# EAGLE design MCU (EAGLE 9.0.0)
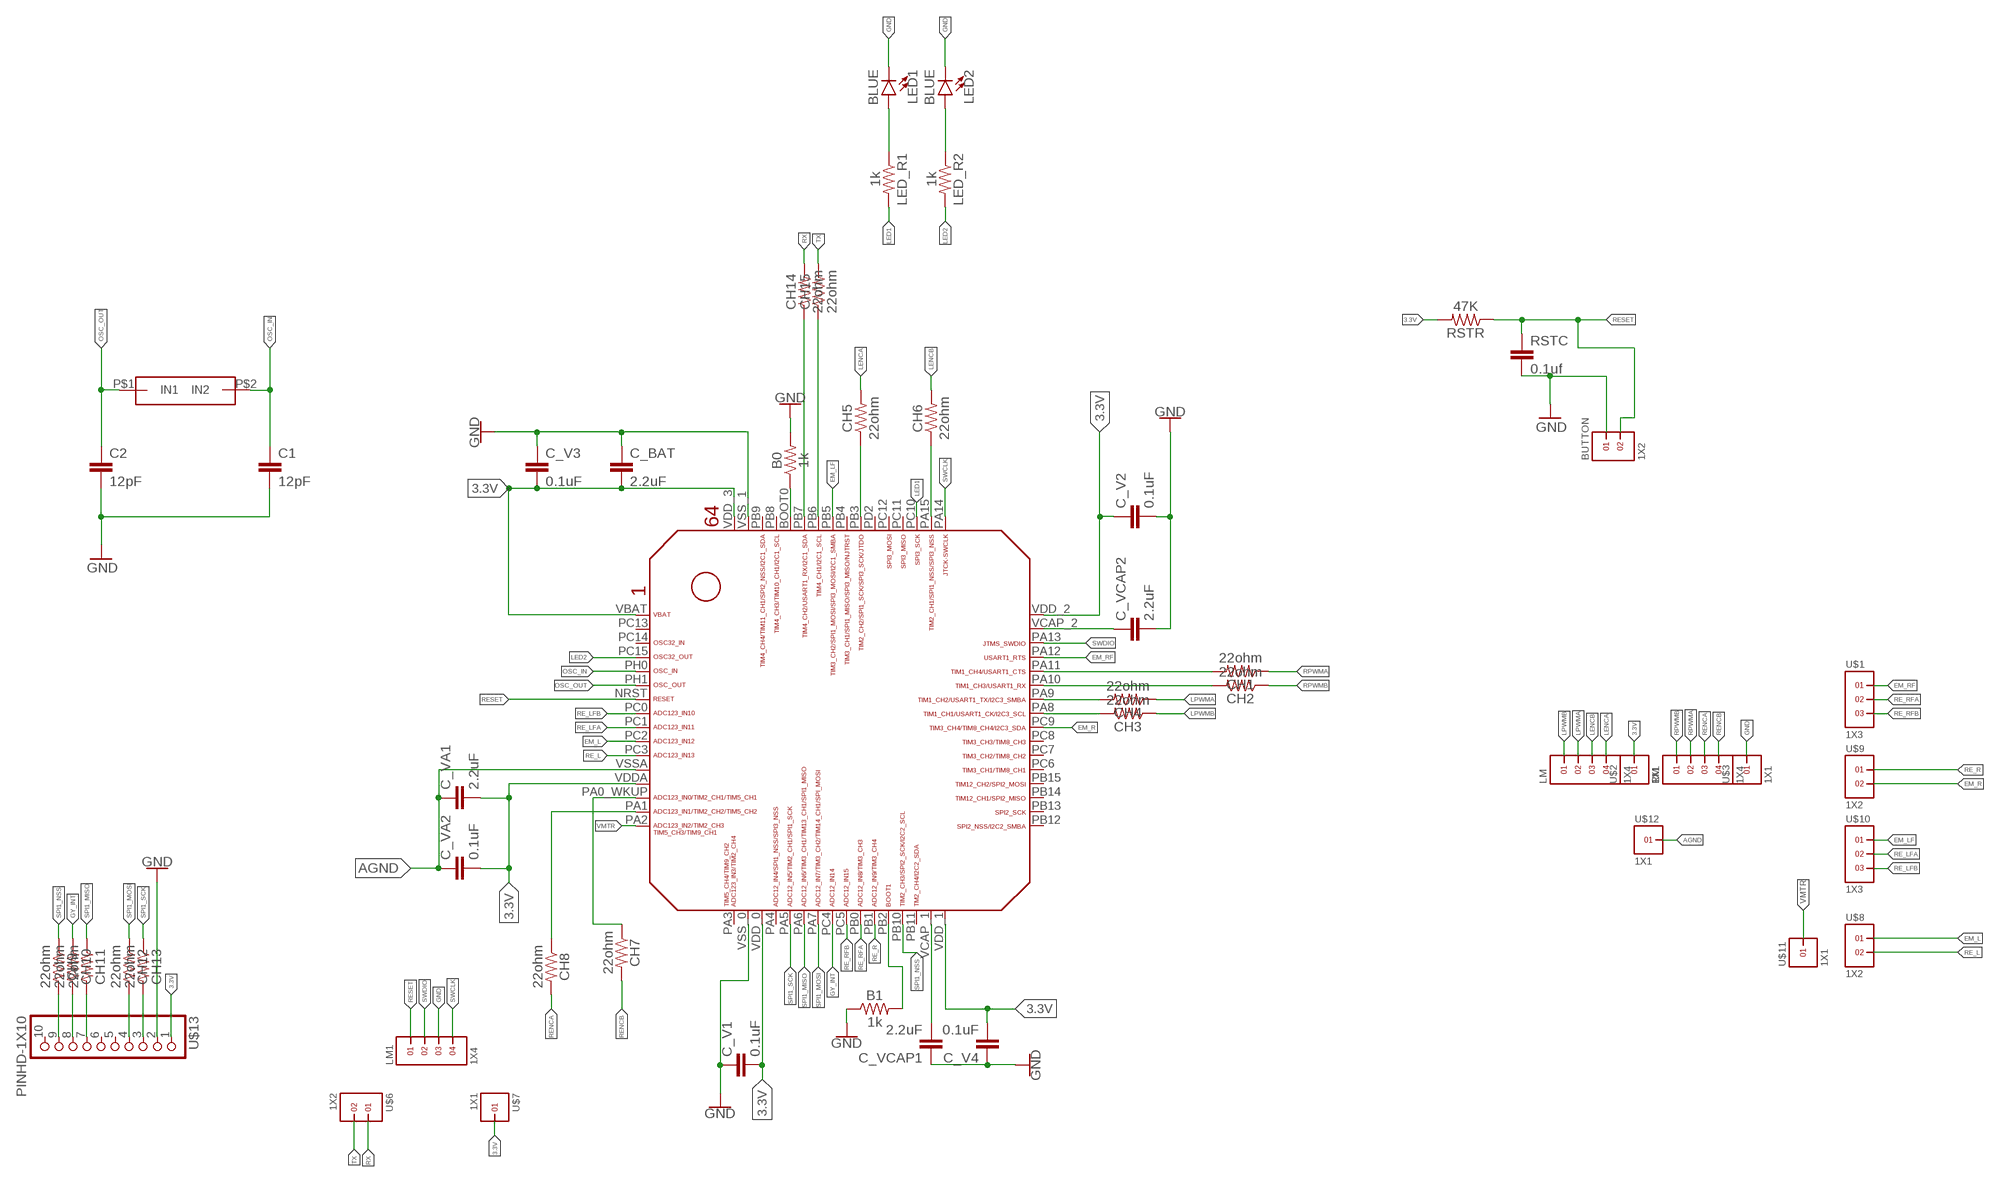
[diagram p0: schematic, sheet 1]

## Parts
B0  1k  0.75OHM-0805-1/4W-1%  [0805]
B1  1k  0.75OHM-0805-1/4W-1%  [0805]
BUTTON  1X2  [1X2]
C1  12pF  22PF-0603-50V-5%  [0603]
C2  12pF  22PF-0603-50V-5%  [0603]
C_BAT  2.2uF  22UF-0805-6.3V-20%  [0805]
C_V1  0.1uF  22UF-0805-6.3V-20%  [0805]
C_V2  0.1uF  22UF-0805-6.3V-20%  [0805]
C_V3  0.1uF  22UF-0805-6.3V-20%  [0805]
C_V4  0.1uF  22UF-0805-6.3V-20%  [0805]
C_VA1  2.2uF  22UF-0805-6.3V-20%  [0805]
C_VA2  0.1uF  22UF-0805-6.3V-20%  [0805]
C_VCAP1  2.2uF  22UF-0805-6.3V-20%  [0805]
C_VCAP2  2.2uF  22UF-0805-6.3V-20%  [0805]
CH1  22ohm  0.75OHM-0805-1/4W-1%  [0805]
CH2  22ohm  0.75OHM-0805-1/4W-1%  [0805]
CH3  22ohm  0.75OHM-0805-1/4W-1%  [0805]
CH4  22ohm  0.75OHM-0805-1/4W-1%  [0805]
CH5  22ohm  0.75OHM-0805-1/4W-1%  [0805]
CH6  22ohm  0.75OHM-0805-1/4W-1%  [0805]
CH7  22ohm  0.75OHM-0805-1/4W-1%  [0805]
CH8  22ohm  0.75OHM-0805-1/4W-1%  [0805]
CH9  22ohm  0.75OHM-0805-1/4W-1%  [0805]
CH10  22ohm  0.75OHM-0805-1/4W-1%  [0805]
CH11  22ohm  0.75OHM-0805-1/4W-1%  [0805]
CH12  22ohm  0.75OHM-0805-1/4W-1%  [0805]
CH13  22ohm  0.75OHM-0805-1/4W-1%  [0805]
CH14  22ohm  0.75OHM-0805-1/4W-1%  [0805]
CH15  22ohm  0.75OHM-0805-1/4W-1%  [0805]
LED1  BLUE  LED-BLUE1206  [LED-1206]
LED2  BLUE  LED-BLUE1206  [LED-1206]
LED_R1  1k  0.75OHM-0805-1/4W-1%  [0805]
LED_R2  1k  0.75OHM-0805-1/4W-1%  [0805]
LM  1X4  [1X4]
LM1  1X4  [1X4]
RM  1X4  [1X4]
RSTC  0.1uf  22UF-0805-6.3V-20%  [0805]
RSTR  47K  0.75OHM-0805-1/4W-1%  [0805]
U$1  1X3  [1X3]
U$2  1X1  [1X1]
U$3  1X1  [1X1]
U$4  STM32F405/415_LQFP64  [STM32F405/415_LQFP64]
U$5  OSC  [OSC]
U$6  1X2  [1X2]
U$7  1X1  [1X1]
U$8  1X2  [1X2]
U$9  1X2  [1X2]
U$10  1X3  [1X3]
U$11  1X1  [1X1]
U$12  1X1  [1X1]
U$13  PINHD-1X10  [1X10-BIG]

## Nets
3.3V: C_BAT.2 C_V1.2 C_V2.1 C_V3.2 C_V4.2 C_VA1.2 C_VA2.2 RSTR.2 U$2.1 U$4.VBAT U$4.VDD_0 U$4.VDD_1 U$4.VDD_2 U$4.VDD_3 U$4.VDDA U$7.1 U$13.1
AGND: C_VA1.1 C_VA2.1 U$4.VSSA U$12.1
EM_L: U$4.PC2 U$8.1
EM_LF: U$4.PB5 U$10.1
EM_R: U$4.PC9 U$9.2
EM_RF: U$1.1 U$4.PA12
GND: B0.2 B1.1 BUTTON.1 C1.2 C2.2 C_BAT.1 C_V1.1 C_V2.2 C_V3.1 C_V4.1 C_VCAP1.1 C_VCAP2.2 LED1.C LED2.C LM1.3 RSTC.2 U$3.1 U$4.VSS_0 U$4.VSS_1 U$13.2
GY_INT: CH10.1 U$4.PC4
INT: CH10.2 U$13.8
LED1: LED_R1.2 U$4.PC10
LED2: LED_R2.2 U$4.PC15
LENCA: CH5.2 LM.4
LENCB: CH6.2 LM.3
LPWMA: CH4.1 LM.2
LPWMB: CH3.1 LM.1
MISO: CH11.2 U$13.7
MOSI: CH12.2 U$13.4
N$1: CH3.2 U$4.PA8
N$2: CH4.2 U$4.PA9
N$3: CH1.2 U$4.PA11
N$4: CH2.2 U$4.PA10
N$5: CH6.1 U$4.PA15
N$6: CH5.1 U$4.PB3
N$7: CH7.1 U$4.PA0_WKUP(PA0_AKUP)
N$8: CH8.1 U$4.PA1
N$9: B1.2 U$4.PB2
N$10: B0.1 U$4.BOOT0
N$11: CH14.1 U$4.PB7
N$12: CH15.1 U$4.PB6
N$13: LED2.A LED_R2.1
N$14: LED1.A LED_R1.1
NSS: CH9.2 U$13.9
OSC_IN: C1.1 U$4.PH0 U$5.P$2(IN2)
OSC_OUT: C2.1 U$4.PH1 U$5.P$1(IN1)
RE_L: U$4.PC3 U$8.2
RE_LFA: U$4.PC1 U$10.2
RE_LFB: U$4.PC0 U$10.3
RE_R: U$4.PB1 U$9.1
RE_RFA: U$1.2 U$4.PB0
RE_RFB: U$1.3 U$4.PC5
RENCA: CH8.2 RM.3
RENCB: CH7.2 RM.4
RESET: BUTTON.2 LM1.1 RSTC.1 RSTR.1 U$4.NRST
RPWMA: CH1.1 RM.2
RPWMB: CH2.1 RM.1
RX: CH14.2 U$6.1
SCK: CH13.2 U$13.3
SPI1_MISO: CH11.1 U$4.PA6
SPI1_MOSI: CH12.1 U$4.PA7
SPI1_NSS: CH9.1 U$4.PB10
SPI1_SCK: CH13.1 U$4.PA5
SWCLK: LM1.4 U$4.PA14
SWDIO: LM1.2 U$4.PA13
TX: CH15.2 U$6.2
VCAP_1: C_VCAP1.2 U$4.VCAP_1
VCAP_2: C_VCAP2.1 U$4.VCAP_2
VMTR: U$4.PA2 U$11.1
Unconnected: U$4.PA3 U$4.PA4 U$4.PB4 U$4.PB8 U$4.PB9 U$4.PB11 U$4.PB12 U$4.PB13 U$4.PB14 U$4.PB15 U$4.PC6 U$4.PC7 U$4.PC8 U$4.PC11 U$4.PC12 U$4.PC13 U$4.PC14 U$4.PD2 U$13.5 U$13.6 U$13.10

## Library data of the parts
B0 B1 CH1-CH15 LED_R1 LED_R2 RSTR = SparkFun-Resistors:0.75OHM: 0.75Ω resistor; PROD_ID: RES-08474; VALUE: 0.75
BUTTON U$6 U$8 U$9 = headers(2mm):1X2
C1 C2 = SparkFun-Capacitors:22PF: 22pF ceramic capacitors; PROD_ID: CAP-07876; VALUE: 22pF
C_BAT C_V1-C_V4 C_VA1 C_VA2 C_VCAP1 C_VCAP2 RSTC = SparkFun-Capacitors:22UF: 22µF ceramic capacitors; PROD_ID: CAP-08402; VALUE: 22uF
LED1 LED2 = SparkFun-LED:LED-BLUE: Blue SMD LED; PROD_ID: DIO-09911
LM LM1 RM = headers(2mm):1X4
U$1 U$10 = headers(2mm):1X3
U$2 U$3 U$7 U$11 U$12 = headers(2mm):1X1
U$4 = STM32F405RG:STM32F405/415_LQFP64
U$5 = Cristal Oscillator:OSC
U$13 = adafruit:PINHD-1X10: Pin header 1x10 0.1" spacing With round pins

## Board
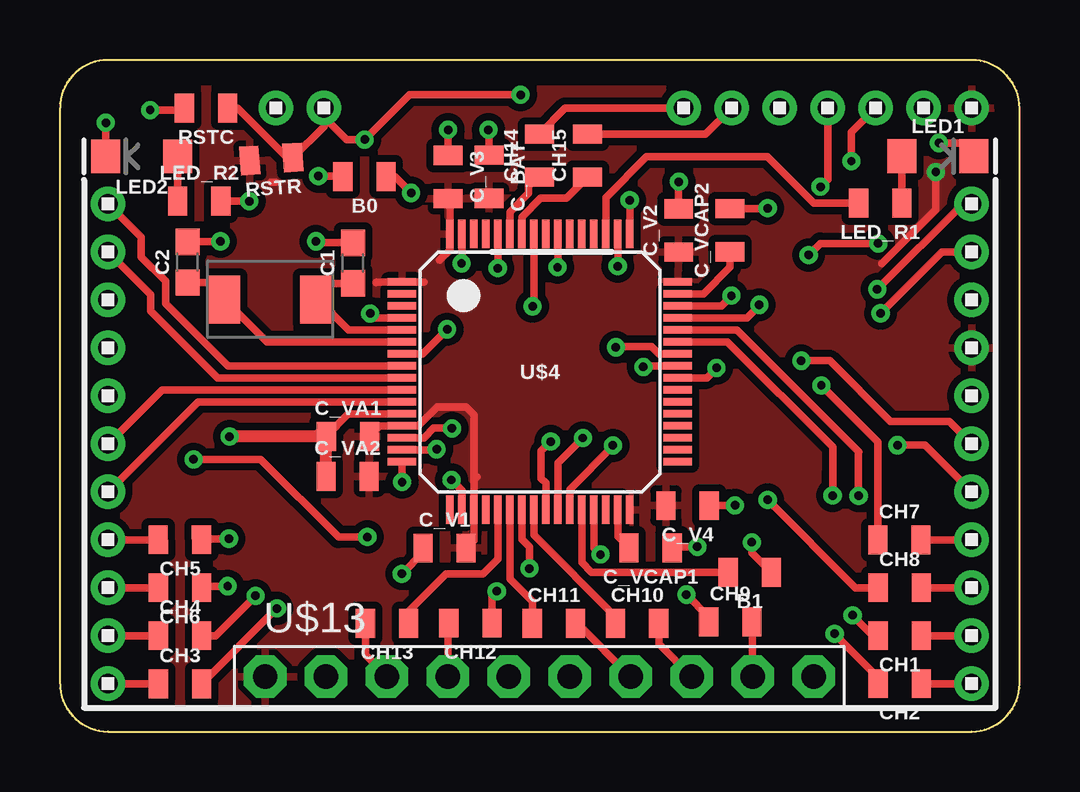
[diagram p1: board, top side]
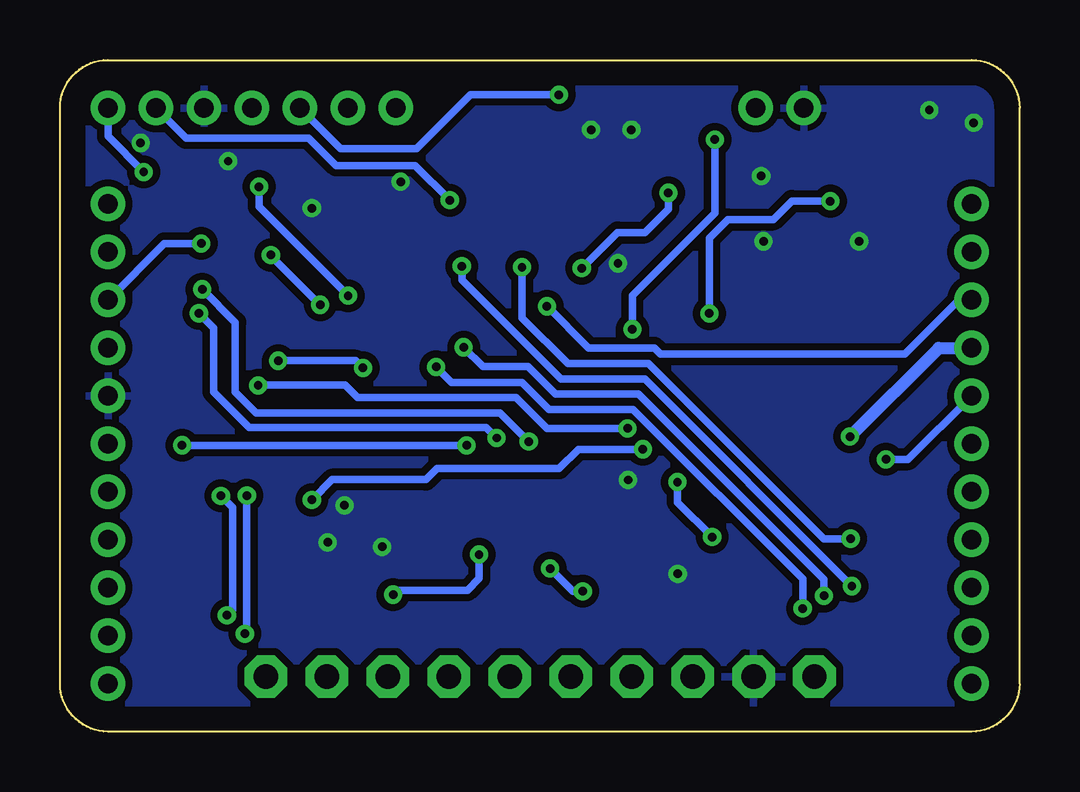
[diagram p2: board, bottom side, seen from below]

Size 40 x 28 mm. Coordinates in mm from the lower left corner, seen from the top.
Outline: 0,2 0,26 arc-90 2,28 38,28 arc-90 40,26 40,2 arc-90 38,0 2,0 arc-90 0,2
Copper layers (1*16): Top 0.035mm / dielectric 1.5mm / Bottom 0.035mm
Design rules "default": minimum track width 6mil, minimum drill 0.35mm, track to track 6mil, track to pad 6mil, pad to pad 6mil, via to via 6mil, smd to smd 6mil, copper to edge 40mil, drill to drill 6mil, minimum pad ring 10mil, minimum via ring 8mil, stop-mask expansion 4mil, vias tented up to drill 0mil, thermal gap 10mil

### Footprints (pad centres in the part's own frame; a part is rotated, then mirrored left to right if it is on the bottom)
0805 = smd 0.8 x 1.2: 1 -0.9,0; 2 0.9,0
1X2 = drill 0.8 pad 1.422: 1 -1,0; 2 1,0
0603 = smd 1.1 x 1: 1 -0.85,0; 2 0.85,0
LED-1206 = smd 1.2 x 1.4: A -1.5,0; C 1.5,0
1X4 = drill 0.8 pad 1.422: 1 -3,0; 2 -1,0; 3 1,0; 4 3,0
1X3 = drill 0.8 pad 1.422: 1 -2,0; 2 0,0; 3 2,0
1X1 = drill 0.8 pad 1.422: 1 0,0
STM32F405/415_LQFP64 = smd 0.3 x 1.2: BOOT0 -1.75,5.75; PA3 -3.75,-5.75; PA4 -2.25,-5.75; PA5 -1.75,-5.75; PA6 -1.25,-5.75; PA7 -0.75,-5.75; PA14 3.75,5.75; PA15 3.25,5.75; PB0 0.75,-5.75; PB1 1.25,-5.75; PB2 1.75,-5.75; PB3 0.75,5.75; PB4 0.25,5.75; PB5 -0.25,5.75; PB6 -0.75,5.75; PB7 -1.25,5.75; PB8 -2.25,5.75; PB9 -2.75,5.75; PB10 2.25,-5.75; PB11 2.75,-5.75; PC4 -0.25,-5.75; PC5 0.25,-5.75; PC10 2.75,5.75; PC11 2.25,5.75; PC12 1.75,5.75; PD2 1.25,5.75; VCAP_1 3.25,-5.75; VDD_0 -2.75,-5.75; VDD_1 3.75,-5.75; VDD_3 -3.75,5.75; VSS_0 -3.25,-5.75; VSS_1 -3.25,5.75 | smd 1.2 x 0.3: NRST -5.75,0.75; PA0_WKUP -5.75,-2.75; PA1 -5.75,-3.25; PA2 -5.75,-3.75; PA8 5.75,0.25; PA9 5.75,0.75; PA10 5.75,1.25; PA11 5.75,1.75; PA12 5.75,2.25; PA13 5.75,2.75; PB12 5.75,-3.75; PB13 5.75,-3.25; PB14 5.75,-2.75; PB15 5.75,-2.25; PC0 -5.75,0.25; PC1 -5.75,-0.25; PC2 -5.75,-0.75; PC3 -5.75,-1.25; PC6 5.75,-1.75; PC7 5.75,-1.25; PC8 5.75,-0.75; PC9 5.75,-0.25; PC13 -5.75,3.25; PC14 -5.75,2.75; PC15 -5.75,2.25; PH0 -5.75,1.75; PH1 -5.75,1.25; VBAT -5.75,3.75; VCAP_2 5.75,3.25; VDD_2 5.75,3.75; VDDA -5.75,-2.25; VSSA -5.75,-1.75
OSC = smd 1.3 x 2: P$1 0,0.1; P$2 3.8,0.1
1X10-BIG = drill 1.016 pad 1.778 octagon: 1 -11.43,0; 2 -8.89,0; 3 -6.35,0; 4 -3.81,0; 5 -1.27,0; 6 1.27,0; 7 3.81,0; 8 6.35,0; 9 8.89,0; 10 11.43,0

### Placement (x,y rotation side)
B0  12.69,23.13 180 top
B1  28.75,6.64 180 top
BUTTON  10,26 0 top
C1  12.21,19.53 90 top
C2  5.32,19.57 90 top
C_BAT  17.88,23.13 270 top
C_V1  16.03,7.65 0 top
C_V2  25.79,20.89 90 top
C_V3  16.18,23.12 270 top
C_V4  26.16,9.42 180 top
C_VA1  12,12.3 0 top
C_VA2  11.99,10.64 0 top
C_VCAP1  24.62,7.66 180 top
C_VCAP2  27.93,20.9 90 top
CH1  35,4 180 top
CH2  35,2 180 top
CH3  5,1.99 0 top
CH4  5,4 0 top
CH5  5,8 180.1 top
CH6  5,6 180 top
CH7  34.99,7.99 0 top
CH8  35,6 0 top
CH9  27.94,4.57 0 top
CH10  24.06,4.51 0 top
CH11  20.59,4.51 0 top
CH12  17.11,4.52 180 top
CH13  13.63,4.51 180 top
CH14  19.99,24.01 90 top
CH15  21.99,24.01 90 top
LED1  36.59,23.99 0 top
LED2  3.41,23.98 180 top
LED_R1  34.19,22.03 180 top
LED_R2  5.81,22.11 0 top
LM  2,5 90 top
LM1  33,26 0 top
RM  38,5 90 top
RSTC  6.09,25.99 180 top
RSTR  8.81,23.87 184.1 top
U$1  38,20 90 top
U$2  38,16 0 top
U$3  38,14 0 top
U$4  20,15 0 top
U$5  6.86,17.92 0 top
U$6  27,26 0 top
U$7  38,26 0 top
U$8  2,11 270 top
U$9  38,11 90 top
U$10  2,20 90 top
U$11  2,14 0 top
U$12  2,16 0 top
U$13  19.98,2.29 0 top

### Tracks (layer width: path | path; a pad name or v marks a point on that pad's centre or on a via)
3.3V  (via drill 0.35)
  Top 0.305: C_V3.2 16.25,22.15 U$4.VDD_3 16.25,20.08 15.82,19.65 | C_VA1.2 13.32,12.75 U$4.VDDA 14.93,12.75 15.16,12.97 15.16,12.98 15.71,13.53 16.92,13.53 17.25,13.2 17.25,10.48 | 17.17,7.89 C_V1.2 17.25,7.97 U$4.VDD_0 17.25,10.48 | 17.25,10.48 17.38,10.61 | U$4.VBAT | U$4.VBAT 15.17,18.74 | U$4.VBAT 13.19,18.74 13.17,18.72 | v36.51,23.33 36.51,21.76 34.26,19.51 | 8.81,22.91 8.99,22.91
  Bottom 0.305: U$7.1 38,24.82 v36.51,23.33
  pour Top (isolate 0.305): -5.02,34.34 47.27,33.34 47.27,-6.7 -5.04,-6.7 -5.04,33.35
AGND  (via drill 0.35)
  Top 0.305: U$4.VSSA 12.02,13.25 C_VA1.1
  Top 0.508: C_VA2.1 C_VA1.1 | 10.7,12.33 C_VA1.1 | C_VA1.1 v7.07,12.3
  Bottom 0.508: v7.07,12.3 3.37,16 U$12.1
EM_L
  Top 0.305: U$8.1 4.25,14.25 U$4.PC2
EM_LF  (via drill 0.35)
  Top 0.305: U$4.PB5 19.75,17.78 v19.7,17.73
  Bottom 0.305: v19.7,17.73 17.96,15.99 15.22,15.99 14.97,15.74 4.79,15.74 2.53,18 U$10.1
EM_R  (via drill 0.35)
  Top 0.305: U$4.PC9 26.96,14.75 v27.37,15.16 | v30.9,15.46 32.09,15.46 34.62,12.93 37.07,12.93 U$9.2
  Bottom 0.305: v27.37,15.16 27.67,15.46 v30.9,15.46
EM_RF  (via drill 0.35)
  Top 0.305: U$4.PA12 28.64,17.25 29.15,17.76 v29.15,17.79 | v31.21,19.87 31.69,20.35 v34.11,20.35
  Bottom 0.305: v29.15,17.79 31.21,19.85 v31.21,19.87 | v34.11,20.35 35.65,20.35 U$1.1
GND  (via drill 0.35)
  Top 0.305: C_V3.1 v16.18,25.09 | U$4.VSS_1 v16.75,19.53 v16.74,19.52 | C_VCAP1.1 25.56,7.7 v26.57,7.7 | C_V4.1 v28.13,9.42 v28.14,9.43 | B1.1 28.84,7.45 v28.84,7.89 | U$4.VSS_0 16.75,10.06 v16.32,10.49 | C_V1.1 15.13,7.46 v14.25,6.58 | C_V2.2 v25.79,22.91 v25.8,22.92 | B0.2 11.76,23.16 v10.77,23.16 | C_BAT.1 17.88,25.07 v17.86,25.09 | C_VCAP2.2 29.48,21.8 v29.5,21.82 | C2.2 6.67,20.42 v6.69,20.44 | C1.2 10.73,20.38 v10.67,20.44 | LM1.3 32.99,24.99 v32.99,23.78 | LED1.C 37.54,24.54 v36.64,24.54 | LED2.C v1.91,25.38 | RSTC.2 5.11,25.91 v3.76,25.91
  pour Bottom (isolate 0.305): -2.47,31.18 -2.47,-3.88 -2.33,-4.02 43.07,-4.02 43.07,31.18 -3.45,32.18 -2.45,31.19
GY_INT
  Top 0.305: U$4.PC4 19.75,8.2 23.16,4.79 CH10.1
INT
  Top 0.305: U$13.8 24.96,3.66 CH10.2
LED1
  Top 0.305: U$4.PC10 22.75,22.27 24.44,23.96 29.49,23.96 31.42,22.03 LED_R1.2
LED2  (via drill 0.35)
  Top 0.305: U$4.PC15 13.11,17.25 v12.93,17.43 | LED_R2.2 6.73,22.11 v7.89,22.11
  Bottom 0.305: v12.93,17.43 12.93,20.58 12.16,21.35 10.27,21.35 9.5,22.12 v7.9,22.12 v7.89,22.11
LENCA
  Top 0.305: LM.4 CH5.2
LENCB
  Top 0.305: LM.3 CH6.2
LPWMA
  Top 0.305: LM.2 CH4.1
LPWMB
  Top 0.305: LM.1 CH3.1
MISO
  Top 0.305: U$13.7 21.57,4.51 CH11.2
MOSI
  Top 0.305: U$13.4 16.17,4.48 CH12.2
N$1  (via drill 0.35)
  Top 0.305: U$4.PA8 24.37,15.25 v24.32,15.2 | v9.04,5.13 CH3.2
  Bottom 0.305: v24.32,15.2 23.68,14.56 20.75,14.56 19.62,13.43 16.11,13.43 9.04,6.36 v9.04,5.13
N$2  (via drill 0.35)
  Top 0.305: U$4.PA9 24.97,15.75 24.66,16.06 23.21,16.06 v23.17,16.02 | v8.15,5.66 6.49,4 CH4.2
  Bottom 0.305: v23.17,16.02 22.36,15.21 20.49,15.21 19.35,14.07 15.88,14.07 8.15,6.34 v8.15,5.66
N$3  (via drill 0.35)
  Top 0.305: v33.04,4.85 33.89,4 CH1.2 | U$4.PA11 28.21,16.75 33.31,11.65 33.29,11.63 v33.29,9.83
  Bottom 0.305: v33.29,9.83 32.81,9.35 32.81,5.08 v33.04,4.85
N$4  (via drill 0.35)
  Top 0.305: v32.29,4.08 34.1,2.27 CH2.2 | v32.21,9.84 32.21,10.66 32.21,10.79 32.21,11.87 27.83,16.25 U$4.PA10
  Bottom 0.305: v32.29,4.08 32.21,4.16 v32.21,9.84
N$5  (via drill 0.35)
  Top 0.305: U$4.PA15 v23.25,19.4 | v6.99,6.06 5.96,6.06 CH6.1
  Bottom 0.305: v23.25,19.4 23.25,18.82 19.12,14.69 15.62,14.69 v6.99,6.06
N$6  (via drill 0.35)
  Top 0.305: U$4.PB3 v20.75,19.37 v20.74,19.36 | 6.17,8 CH5.1 5.94,8.04 v7.04,8.04
  Bottom 0.305: v7.04,8.04 8.16,8.04 15.46,15.34 18.83,15.34 20.74,17.25 v20.74,19.36
N$7  (via drill 0.35)
  Top 0.305: 15.03,12.25 U$4.PA0_WKUP 15.17,12.25 15.57,12.65 v16.33,12.65 v16.34,12.64 | v31.74,14.43 34.09,12.08 CH7.1
  Bottom 0.305: v16.34,12.64 19.7,12.64 20.98,13.92 27.59,13.92 28.11,14.44 v31.73,14.44 v31.74,14.43
N$8  (via drill 0.35)
  Top 0.305: U$4.PA1 15.68,11.75 v15.7,11.77 | v29.5,9.66 33.16,6 CH8.1
  Bottom 0.305: v15.7,11.77 18.39,11.77 19.19,10.97 24.29,10.97 24.75,10.51 28.65,10.51 v29.5,9.66
N$9
  Top 0.305: B1.2 22.16,6.64 21.75,7.05 U$4.PB2
N$10  (via drill 0.35)
  Top 0.305: U$4.BOOT0 v18.25,19.32 | v14.64,22.46 13.97,23.13 B0.1
  Bottom 0.305: v18.25,19.32 16.76,20.81 15.62,20.81 14.64,21.79 v14.64,22.46
N$11
  Top 0.305: U$4.PB7 18.75,21.66 19.54,22.45 19.54,22.73 19.92,23.11 CH14.1
N$12
  Top 0.305: U$4.PB6 19.25,21.45 20.04,22.24 21.12,22.24 CH15.1
N$13
  Top 0.305: LED_R2.1 LED2.A
N$14
  Top 0.305: LED_R1.1 LED1.A
NSS
  Top 0.305: U$13.9 28.87,4.54 CH9.2
OSC_IN
  Top 0.305: C1.1 11.32,18.68 10.71,18.07 | 10.71,18.07 U$5.P$2 | U$4.PH0 12.03,16.75 10.71,18.07
OSC_OUT
  Top 0.305: U$4.PH1 8.63,16.25 U$5.P$1 6.16,18.72 C2.1
RE_L
  Top 0.305: U$8.2 5.75,13.75 U$4.PC3
RE_LFA
  Top 0.305: U$4.PC1 6.57,14.75 3.78,17.54 3.78,18.22 U$10.2
RE_LFB
  Top 0.305: U$10.3 3.39,20.61 3.39,19.79 4.4,18.78 4.4,17.85 7,15.25 U$4.PC0
RE_R  (via drill 0.35)
  Top 0.305: U$4.PB1 21.25,10.1 23.05,11.9 v23.05,11.93 | v34.91,11.94 36.06,11.94 U$9.1
  Bottom 0.305: v23.05,11.93 v34.9,11.93 v34.91,11.94
RE_RFA  (via drill 0.35)
  Top 0.305: v21.8,12.24 20.75,11.19 U$4.PB0 | v34.21,17.44 36.77,20 U$1.2
  Bottom 0.305: v21.8,12.24 22.23,12.67 32.11,12.67 33.6,14.16 33.6,16.83 v34.21,17.44
RE_RFB  (via drill 0.35)
  Top 0.305: U$4.PC5 20.25,10.36 20.06,10.55 20.06,11.69 v20.46,12.09 | v34.07,18.44 37.63,22 U$1.3
  Bottom 0.305: v20.46,12.09 21.66,13.29 31.83,13.29 32.69,14.15 32.69,17.06 v34.07,18.44
RENCA
  Top 0.305: CH8.2 RM.3
RENCB
  Top 0.305: CH7.2 RM.4
RESET  (via drill 0.35)
  Top 0.305: U$4.NRST 15.12,15.75 v16.14,16.77 | v19.2,26.55 14.57,26.55 v12.7,24.68 11.94,24.68 11,25.62 | 9.61,24.23 RSTR.1 | 11,25.62 BUTTON.2 | RSTC.1 7.41,25.99 9.47,23.93 RSTR.1 | RSTR.1 11,25.23 11,25.62
  Bottom 0.305: v16.14,16.77 16.14,18.18 12.7,21.62 v12.7,24.68 | v19.2,26.55 22.88,26.55 25.13,24.3 28.3,24.3 LM1.1
RPWMA
  Top 0.305: CH1.1 RM.2
RPWMB
  Top 0.305: CH2.1 RM.1
RX
  Top 0.305: CH14.2 21.06,25.98 25.98,25.98 U$6.1
SCK
  Top 0.305: U$13.3 12.73,3.19 CH13.2
SPI1_MISO
  Top 0.305: U$4.PA6 18.75,6.37 19.69,5.43 CH11.1
SPI1_MOSI  (via drill 0.35)
  Top 0.305: v18.21,5.85 18.01,5.65 CH12.1 | U$4.PA7 19.25,8.02 19.57,7.7 v19.57,6.8
  Bottom 0.305: v18.21,5.85 18.62,5.85 v19.57,6.8
SPI1_NSS  (via drill 0.35)
  Top 0.305: 27.04,4.82 27.04,4.78 | CH9.1 27.04,4.66 27.04,4.78 | U$4.PB10 22.25,7.66 v22.53,7.38 | v26.11,5.71 27.04,4.78
  Bottom 0.305: v22.53,7.38 22.53,6.38 23.02,5.89 25.93,5.89 v26.11,5.71
SPI1_SCK
  Top 0.305: U$4.PA5 18.25,7.2 17.63,6.58 16.09,6.58 14.53,5.02 CH13.1
SWCLK  (via drill 0.35)
  Top 0.305: U$4.PA14 v23.75,22.15
  Bottom 0.305: v23.75,22.15 25.2,23.6 26.08,23.6 26.09,23.6 28.48,23.6 29.63,24.75 34.75,24.75 LM1.4
SWDIO  (via drill 0.35)
  Top 0.305: U$4.PA13 27.57,17.75 v27.99,18.17 | LM1.2 32,23.01 v31.7,22.71
  Bottom 0.305: v31.7,22.71 31.7,21.88 v27.99,18.17
TX
  Top 0.305: CH15.2 26.91,24.91 U$6.2
VCAP_1
  Top 0.305: U$4.VCAP_1 23.25,8.13 C_VCAP1.2
VCAP_2
  Top 0.305: U$4.VCAP_2 26.82,18.25 27.93,19.36 C_VCAP2.1
VMTR  (via drill 0.35)
  Top 0.305: U$4.PA2 v14.25,10.41 v14.26,10.4 | v12.81,8.11 11.61,8.11 8.37,11.35 v5.57,11.35
  Bottom 0.305: v14.26,10.4 14.26,9.56 v12.81,8.11 | v5.57,11.35 4.65,11.35 U$11.1

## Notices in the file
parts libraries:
SparkFun-PowerSymbols: Licensing: Creative Commons ShareAlike 4.0 International - https://creativecommons.org/licenses/by-sa/4.0
